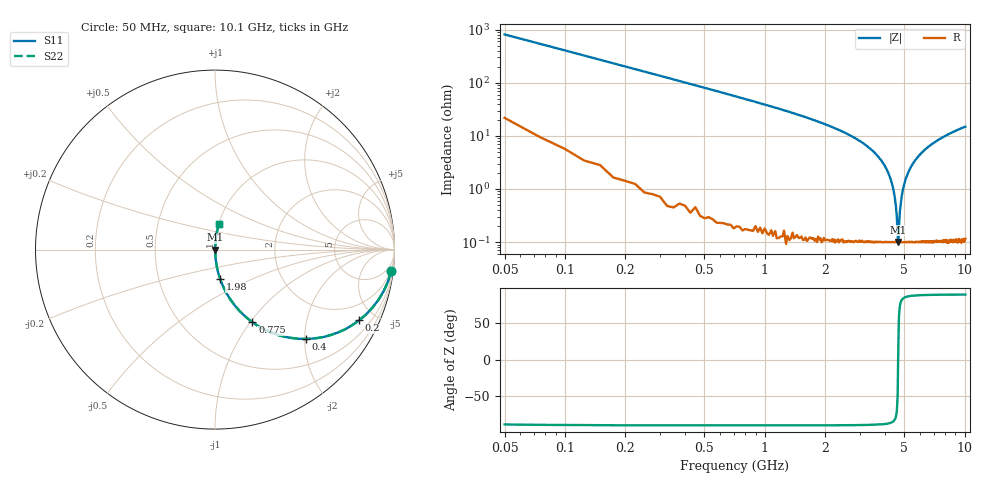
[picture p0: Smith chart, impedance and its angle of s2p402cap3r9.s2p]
! AVX Thin Film Operation		Date: April 2003
! Description: Accu-P® Series, Thin Film, SMD, RF Capacitor
! Part Number: 04025J3R9ABS
! 50 MHz  -  10.05 GHz
! Serial Measurements
# hz S db R 50
!	S11		S21		S12		S22
!	dB	Phase	dB	Phase	dB	Phase	dB	Phase
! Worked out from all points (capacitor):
!   400 points, 50 MHz to 10.1 GHz, reference 50 ohm
!   read as one part in series: C = 3.9 pF near 100 MHz
!   lowest |Z| = 100 mohm at 4.65 GHz (marker M1)
!   series resonance near 4.654 GHz, so ESL is about 300 pH
!   S11 on the Smith chart (normalised r, x): 50 MHz: 1, -16; 200 MHz: 1.03, -4.07; 400 MHz: 1.01, -2.03; 775 MHz: 1.00, -1.02; 1.98 GHz: 1.00, -0.34; 10.1 GHz: 1.00, +0.30
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5e7  -0.09 -7.0  -18.30 81.5  -18.30 81.5  -0.09 -7.0
1e8  -0.28 -13.7  -12.50 75.5  -12.50 75.5  -0.28 -13.7
2e8  -0.96 -26.1  -7.14 63.5  -7.14 63.5  -0.96 -26.1
4e8  -2.97 -44.5  -3.08 45.2  -3.08 45.2  -2.97 -44.5
7.75e8  -6.84 -62.7  -1.02 27.1  -1.02 27.1  -6.84 -62.7
1.73e9  -14.00 -78.2  -0.19 11.5  -0.19 11.5  -14.00 -78.2
1.98e9  -15.60 -80.0  -0.13 9.6  -0.13 9.6  -15.60 -80.0
3.4e9  -25.10 -85.8  -0.02 3.2  -0.02 3.2  -25.10 -85.8
3.98e9  -31.10 -86.3  -0.01 1.6  -0.01 1.6  -31.10 -86.3
4.33e9  -37.80 -84.8  -0.01 0.7  -0.01 0.7  -37.80 -84.8
4.53e9  -46.00 -78.2  -0.01 0.3  -0.01 0.3  -46.00 -78.2
4.58e9  -50.10 -71.2  -0.01 0.2  -0.01 0.2  -50.10 -71.2
4.65e9  -60.00 -6.3  -0.01 0.0  -0.01 0.0  -60.00 -6.3
4.68e9  -57.70 39.6  -0.01 -0.0  -0.01 -0.0  -57.70 39.6
4.75e9  -48.50 74.4  -0.01 -0.2  -0.01 -0.2  -48.50 74.4
4.8e9  -45.10 79.3  -0.01 -0.3  -0.01 -0.3  -45.10 79.3
4.9e9  -40.80 83.2  -0.01 -0.5  -0.01 -0.5  -40.80 83.2
5.08e9  -36.30 85.4  -0.01 -0.9  -0.01 -0.9  -36.30 85.4
5.7e9  -28.90 86.3  -0.01 -2.0  -0.01 -2.0  -28.90 86.3
6.75e9  -23.50 85.3  -0.03 -3.8  -0.03 -3.8  -23.50 85.3
8.43e9  -19.20 83.2  -0.06 -6.3  -0.06 -6.3  -19.20 83.2
1.01e10  -16.70 81.1  -0.10 -8.5  -0.10 -8.5  -16.70 81.1
